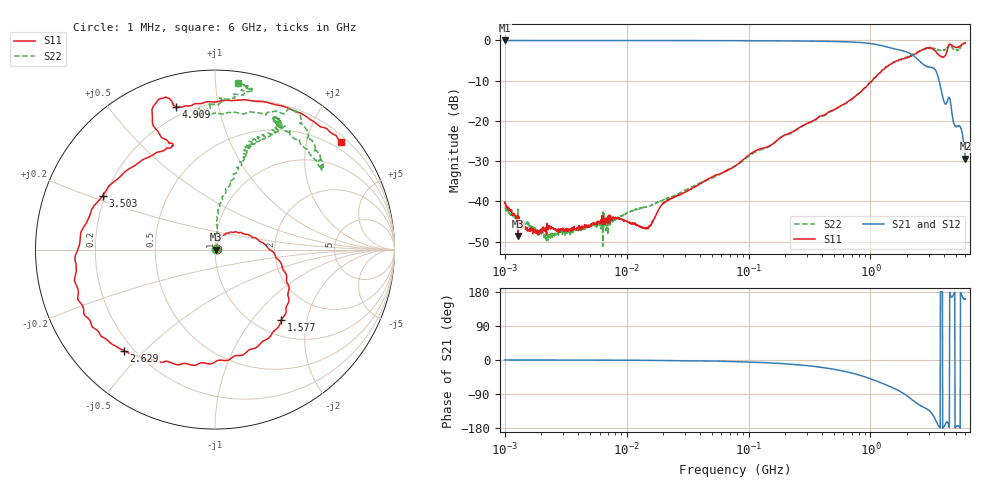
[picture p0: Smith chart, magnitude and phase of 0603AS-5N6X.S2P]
!s-Parameter Generated by FASTRON Sdn. Bhd.
!FASTRON P/N : 0603AS-5N6X
!Keysight Technologies: E5071C_MY46733604_B.14.02
!Date: Tue Nov 21 15:07:36 2023
!Version  :Rev01  Tue Nov 21 15:07:36 2023
!Data & Calibration Information:
!Freq  S11:SOLT2(ON)  S21:SOLT2(ON)  S12:SOLT2(ON)  S22:SOLT2(ON)
!PortZ  Port1:50+j0  Port2:50+j0
!When reading reference impedance value at option line is always used.
! Remarks : This data is being provided solely for informational purposes.
# Hz S dB R 50
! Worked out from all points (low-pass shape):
!   1601 points, 1 MHz to 6 GHz, reference 50 ohm
!   highest |S21| = -0.03 dB at 1.006 MHz (marker M1); lowest = -29.4 dB at 6 GHz (marker M2)
!   |S21| within 3 dB of the highest: start of sweep to 2.02 GHz
!   lowest |S11| = -48.6 dB at 1.288 MHz (marker M3), VSWR 1.01, Z = 50.4 - j0.00182 ohm
!   |S11| at or under -10 dB: start of sweep to 1.032 GHz
!   |S22| runs from -51.1 to -0.5 dB; largest |S21 - S12| = 0.01
!   S11 on the Smith chart (normalised r, x): 1 MHz: 1.02, +0.01; 1.577 GHz: 1.29, -1.42; 2.629 GHz: 0.17, -0.44; 3.503 GHz: 0.19, +0.22; 4.909 GHz: 0.15, +0.75; 6 GHz: 0.33, +2.69
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1000000  -40.46 18.6  -0.04 0.1  -0.06 0.2  -41.54 23.2
1006392  -40.13 17.5  -0.03 0.1  -0.05 0.2  -41.56 20.3
1287650  -48.61 -0.3  -0.05 0.1  -0.04 -0.0  -41.94 4.1
2190642  -46.75 27.3  -0.05 -0.1  -0.05 -0.1  -48.30 41.1
4277066  -46.77 32.1  -0.05 -0.2  -0.05 -0.2  -47.07 39.3
8079992  -43.96 43.1  -0.05 -0.5  -0.05 -0.5  -44.68 44.6
1.459489e7  -46.70 53.9  -0.05 -0.8  -0.06 -0.8  -41.27 41.9
1.823719e7  -42.17 54.8  -0.05 -1.0  -0.06 -1.0  -40.16 53.8
7.757876e7  -31.24 67.4  -0.08 -4.0  -0.09 -4.0  -31.23 70.1
3.307917e8  -20.09 56.4  -0.20 -16.2  -0.20 -16.2  -20.31 82.7
8.457976e8  -12.58 16.1  -0.56 -41.7  -0.56 -41.7  -12.54 83.6
1.414819e9  -6.18 -33.3  -1.76 -69.0  -1.76 -69.0  -6.21 72.7
1.576786e9  -5.38 -46.5  -2.09 -75.5  -2.10 -75.6  -5.41 73.8
2.098753e9  -4.01 -90.5  -3.22 -100.2  -3.24 -100.3  -3.91 69.0
2.628843e9  -2.42 -132.0  -5.64 -121.7  -5.63 -121.6  -2.39 63.8
3.141603e9  -2.00 -164.2  -6.65 -139.0  -6.61 -139.1  -2.11 64.7
3.502967e9  -3.18 154.3  -8.15 -165.3  -8.13 -165.6  -2.33 56.9
3.887702e9  -4.06 115.4  -13.68 179.8  -13.68 179.5  -2.45 38.8
4.171191e9  -3.33 114.8  -15.76 -165.6  -15.78 -166.0  -2.06 44.4
4.908786e9  -1.69 105.2  -21.16 178.7  -21.20 178.6  -2.42 86.8
5.244544e9  -1.67 92.2  -21.26 -173.2  -21.31 -173.2  -2.27 99.4
6e9  -0.69 40.3  -29.38 160.9  -29.35 161.0  -0.54 82.2
